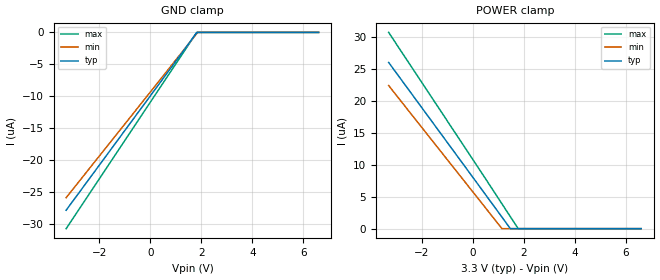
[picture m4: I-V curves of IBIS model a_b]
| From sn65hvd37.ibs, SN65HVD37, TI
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|   a_b Model
[Model]   a_b
Model_type   Input
Vinl = 0.8
Vinh = 2
|   typ   min   max
|   (nom PVT)   (fast PVT)   (slow PVT)
|C_comp from frequency sweep method (F=10MHz)
|Average
|C_comp   3.624e-12   3.545e-12   3.721e-12
|C_comp from LC tank measurement(L=20nH)
|Average
|Resonant Frequency(Hz)   5.770e+09   5.890e+09   5.550e+09
|C_comp   0.76160e-12   0.73089e-12   0.82318e-12
C_comp   2.6e-12   2.6e-12   2.6e-12
| Where nom  PVT is Nominal Process, 3.3V, 27C
|   Fast PVT is Strong Process,  3.6V, -40C
|   Slow PVT is Weak Process,   3V, 125C
[Voltage Range]   3.3   3   3.6
|Ambient Temperature   25   85   -40
|Junction Temperature
[Temperature Range]   27   125   -40
[Power Clamp Reference]   3.3   3   3.6
[GND Clamp Reference]   0   0   0
[GND Clamp]
|   Voltage   I(typ)   I(min)   I(max)
-3.3V     -27.9uA    -25.94uA   -30.8uA
1.818V    -50.29nA   -198.6nA   -10.36nA
1.857V    -11.34nA   0A         0A
6.6V      0A         0A         0A
[POWER Clamp]
|   Voltage   I(typ)   I(min)   I(max)
-3.3V     25.96uA    22.36uA    30.65uA
1.14V     1.82uA     13.16nA    3.893uA
1.472V    0A         0A         1.872uA
1.778V    0A         0A         11.43nA
6.6V      0A         0A         0A
